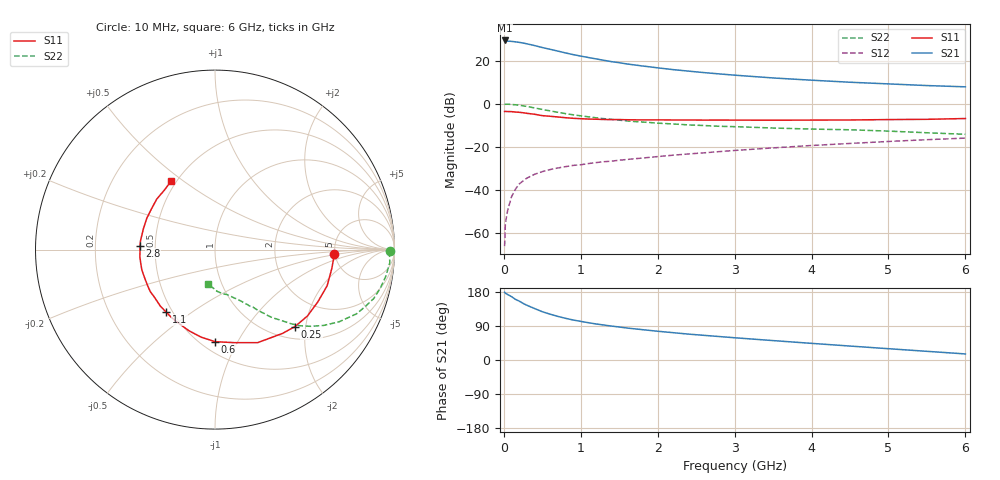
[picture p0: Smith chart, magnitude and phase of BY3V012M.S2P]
! SIEMENS Small Signal Semiconductors
! BFY420
! Si NPN RF SIEGET Grounded Emitter Transistor in MICRO-X
! VCE = 3 V  IC = 12 mA
! Common Emitter S-Parameters:  October  1996
# GHz  S  MA  R  50
!  f  S11  S21  S12  S22
! GHz  MAG  ANG  MAG  ANG  MAG  ANG  MAG  ANG
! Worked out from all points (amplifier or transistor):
!   36 points, 10 MHz to 6 GHz, reference 50 ohm
!   highest |S21| = 29.3 dB at 10 MHz (marker M1)
!   |S21| within 3 dB of that: start of sweep to 468.6 MHz
!   unconditionally stable (mu >= 1): start of sweep to 10.89 MHz; 2.389 GHz to end of sweep
!   at 250 MHz: K = 0.23, MSG = 32.0 dB, |S12| = -35.8 dB
!   at 1.4 GHz: K = 0.80, MSG = 23.1 dB, |S12| = -26.6 dB
!   at 6 GHz: K = 1.08, MAG = 10.1 dB, |S12| = -15.9 dB
!   S11 on the Smith chart (normalised r, x): 10 MHz: 4.90, -0.40; 250 MHz: 1.26, -1.75; 600 MHz: 0.58, -0.81; 1.1 GHz: 0.46, -0.40; 2.8 GHz: 0.41, +0.02; 6 GHz: 0.47, +0.45
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0.01  0.6631 -2.0  29.31 178.8  0.0005 70.4  0.9741 -0.6
0.02  0.6632 -3.6  29.23 176.3  0.0017 80.2  0.9723 -1.5
0.05  0.6595 -9.0  28.29 172.7  0.0034 81.9  0.9767 -4.3
0.1  0.6565 -17.9  27.9 167.2  0.007 80.4  0.9631 -8.9
0.15  0.6427 -27.0  27.2 160.2  0.0104 76.7  0.9455 -13.2
0.2  0.6341 -35.7  26.47 155.4  0.0138 73.1  0.925 -17.2
0.25  0.6184 -43.9  25.54 149.4  0.0163 69.5  0.8939 -20.9
0.3  0.5997 -51.1  24.5 144.4  0.0189 68.5  0.866 -24.4
0.4  0.5703 -65.4  22.32 135.8  0.0232 63.3  0.7999 -30.2
0.5  0.5299 -78.1  20.07 127.4  0.0267 59.8  0.7384 -34.9
0.6  0.5131 -89.9  18.31 121.0  0.0298 57.0  0.6837 -38.7
0.8  0.4749 -107.8  15.09 110.1  0.0348 53.5  0.591 -44.3
0.9  0.4601 -114.7  13.78 105.6  0.0372 52.9  0.555 -46.1
1.1  0.442 -128.1  11.79 98.4  0.0411 52.5  0.4975 -49.8
1.3  0.4318 -138.7  10.17 92.3  0.0453 51.9  0.4517 -52.2
1.6  0.4258 -151.7  8.369 84.4  0.0511 51.4  0.4001 -55.6
2.2  0.4206 -169.5  6.182 72.1  0.0642 51.0  0.3403 -61.2
2.8  0.4186 177.0  4.916 61.9  0.0777 49.1  0.3003 -66.0
3.5  0.4155 163.7  3.961 51.2  0.0948 46.0  0.2739 -71.5
4.5  0.4206 147.1  3.152 36.8  0.1202 39.6  0.2492 -80.4
5.5  0.4357 130.0  2.639 22.9  0.1469 31.5  0.2126 -93.4
6  0.4543 122.4  2.467 16.0  0.1598 27.0  0.1958 -102.1
